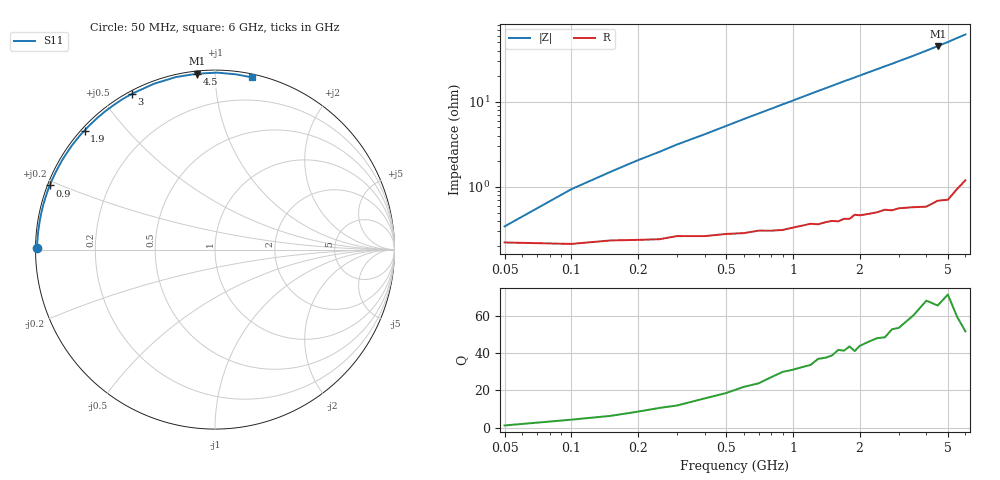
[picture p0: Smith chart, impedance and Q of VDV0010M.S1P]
! Infineon Technologies  Discrete & RF Semiconductors
! BBY 55-03
! Si Tuning Diode in SOD323
! VR =
! S-Parameters:  June  1999
# GHz  S  MA  R  50
!  f  S11
! GHz  MAG  ANG
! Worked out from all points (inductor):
!   34 points, 50 MHz to 6 GHz, reference 50 ohm
!   read as one part to ground: L = 1.57 nH near 100 MHz
!   highest Q = 68.2 at 4.5 GHz (marker M1), where L = 1.6 nH
!   S11 on the Smith chart (normalised r, x): 50 MHz: 0.00, +0.01; 900 MHz: 0.01, +0.19; 1.9 GHz: 0.01, +0.39; 3 GHz: 0.01, +0.60; 4.5 GHz: 0.01, +0.90; 6 GHz: 0.02, +1.24
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0.05  0.9911 179.4
0.1  0.9915 177.9
0.2  0.9905 175.3
0.25  0.9903 174.1
0.3  0.9895 172.8
0.4  0.9896 170.5
0.6  0.9888 165.7
0.8  0.9881 161.1
0.9  0.988 158.8
1  0.9873 156.6
1.1  0.9867 154.3
1.3  0.9865 149.9
1.6  0.9859 143.6
1.7  0.985 141.5
1.8  0.9852 139.6
1.9  0.9837 137.6
2  0.9842 135.7
2.2  0.984 131.9
2.4  0.9838 128.3
2.6  0.9832 124.7
2.8  0.984 121.4
3  0.9836 118.0
3.5  0.9846 110.2
4  0.9858 102.7
4.5  0.9849 95.8
5  0.9861 89.4
5.5  0.9835 83.2
6  0.9813 77.8
